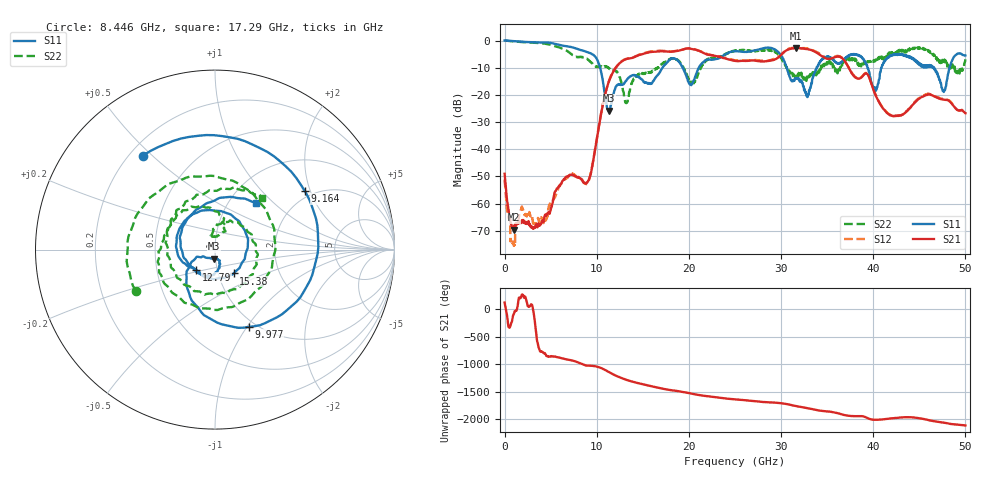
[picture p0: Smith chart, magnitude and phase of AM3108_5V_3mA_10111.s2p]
# Hz S DB R 50.0
!freq dBS11 angS11 dBS21 angS21 dBS12 angS12 dBS22 angS22
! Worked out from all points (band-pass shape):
!   1601 points, 10 MHz to 50 GHz, reference 50 ohm
!   highest |S21| = -2.75 dB at 31.66 GHz (marker M1); lowest = -69.6 dB at 978.6 MHz (marker M2)
!   |S21| within 3 dB of the highest: 14.28 GHz to 22.99 GHz (8.702 GHz wide, 46.7 % of centre); 29.87 GHz to 34.45 GHz (4.58 GHz wide, 14.2 % of centre)
!   lowest |S11| = -25.8 dB at 11.29 GHz (marker M3), VSWR 1.11, Z = 49 - j5 ohm
!   |S11| at or under -10 dB: 10.37 GHz to 17.14 GHz (6.772 GHz wide, 49.2 % of centre); 19.32 GHz to 21.07 GHz (1.753 GHz wide, 8.68 % of centre); 30.62 GHz to 33.85 GHz (3.225 GHz wide, 10 % of centre)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
!   |S22| runs from -23.0 to 0.1 dB; largest |S21 - S12| = 0.024
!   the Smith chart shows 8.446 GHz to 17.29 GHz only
!   S11 on the Smith chart (normalised r, x): 8.446 GHz: 0.25, +0.47; 9.164 GHz: 1.81, +1.83; 9.977 GHz: 0.92, -1.02; 12.79 GHz: 0.79, -0.18; 15.38 GHz: 1.18, -0.32; 17.29 GHz: 1.33, +0.78
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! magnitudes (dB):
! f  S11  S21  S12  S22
! 10 MHz  0.0  -49.0  -51.2  0.1
! 978.6 MHz  -0.2  -69.6  -74.0  -0.3
! 1.853 GHz  -0.4  -67.2  -61.6  -0.5
! 4.384 GHz  -0.7  -64.3  -66.3  -1.1
! 8.352 GHz  -3.5  -51.2  -51.0  -6.0
! 8.446 GHz  -3.6  -51.6  -51.3  -6.1
! 9.164 GHz  -4.5  -51.1  -51.3  -7.3
! 9.977 GHz  -6.6  -36.9  -36.9  -9.7
! 11.29 GHz  -25.8  -15.4  -15.2  -10.1
! 12.79 GHz  -16.3  -7.5  -7.4  -16.9
! 15.38 GHz  -15.5  -4.5  -4.4  -12.1
! 16.69 GHz  -12.3  -4.0  -3.7  -10.0
! 17.29 GHz  -9.2  -3.9  -3.8  -8.2
! 20.41 GHz  -15.4  -3.2  -2.9  -16.0
! 25 GHz  -3.9  -7.5  -7.3  -3.8
! 31.66 GHz  -13.9  -2.7  -2.7  -13.8
! 33.35 GHz  -15.5  -3.5  -3.4  -12.7
! 38 GHz  -4.9  -13.5  -13.3  -6.6
! 40.22 GHz  -18.7  -19.8  -19.7  -7.6
! 41.69 GHz  -6.0  -27.2  -27.0  -5.2
! 47.66 GHz  -18.9  -21.8  -21.6  -7.7
! 50 GHz  -5.5  -26.7  -26.5  -6.9
